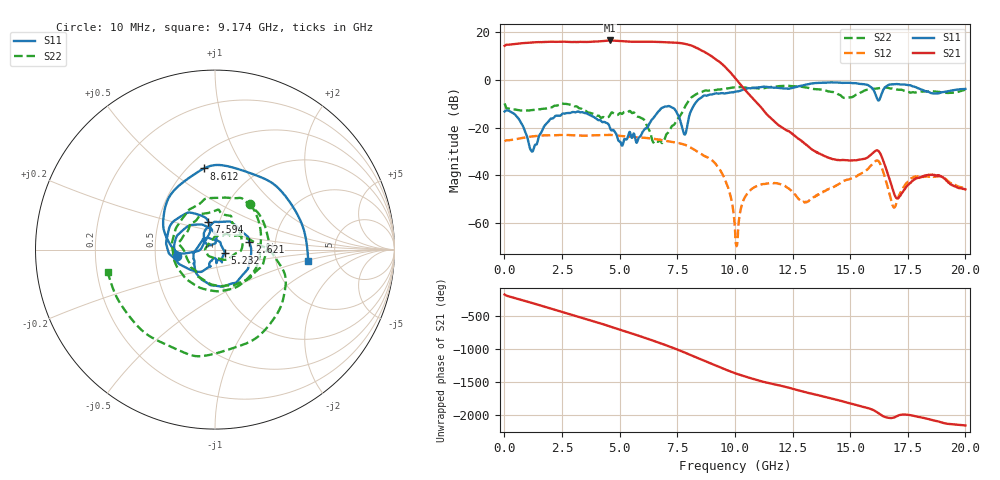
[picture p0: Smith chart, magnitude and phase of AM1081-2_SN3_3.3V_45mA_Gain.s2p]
!Agilent Technologies,E8364B,MY43040894,A.07.50.67
!Agilent E8364B: A.07.50.67
!Date: Wednesday, June 23, 2021 08:05:39
!Correction: S11(Full 2 Port(1,2))
!S21(Full 2 Port(1,2))
!S12(Full 2 Port(1,2))
!S22(Full 2 Port(1,2))
!S2P File: Measurements: S11, S21, S12, S22:
# Hz S  dB  R 50
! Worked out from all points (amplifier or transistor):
!   3201 points, 10 MHz to 20 GHz, reference 50 ohm
!   highest |S21| = 16.6 dB at 4.595 GHz (marker M1)
!   |S21| within 3 dB of that: start of sweep to 8.292 GHz
!   unconditionally stable (mu >= 1): start of sweep to end of sweep
!   at 3.34 GHz: K = 1.21, MAG = 17.0 dB, |S12| = -23.4 dB
!   at 10.01 GHz: K = 214.87, MAG = 5.5 dB, |S12| = -62.7 dB
!   at 20 GHz: K = 6787.26, MAG = -41.5 dB, |S12| = -45.6 dB
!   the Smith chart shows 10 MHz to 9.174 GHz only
!   S11 on the Smith chart (normalised r, x): 10 MHz: 0.65, -0.05; 2.621 GHz: 1.47, +0.13; 5.232 GHz: 1.11, -0.04; 7.594 GHz: 0.89, +0.28; 8.612 GHz: 0.59, +0.68; 9.174 GHz: 3.09, -0.52
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1e7  -13.25 -169.9  14.33 -169.4  -25.75 11.8  -9.86 52.2
6.221938e8  -16.34 115.7  15.30 121.3  -24.68 -46.8  -12.69 -88.1
1.078216e9  -27.72 82.6  15.65 74.8  -23.89 -86.8  -12.82 -147.2
1.846581e9  -18.10 114.3  16.01 -5.2  -23.25 -159.8  -11.96 133.6
2.621194e9  -14.15 12.6  16.06 -86.7  -23.10 125.7  -10.03 44.4
3.345831e9  -13.53 -75.0  16.02 -162.2  -23.38 55.5  -12.12 -41.9
3.883062e9  -15.58 -129.7  16.12 142.0  -23.25 4.3  -14.43 -100.5
4.264122e9  -17.74 -153.6  16.32 101.0  -23.14 -33.8  -15.58 -142.4
4.595206e9  -20.48 168.5  16.60 63.3  -23.10 -68.8  -14.53 175.5
5.232388e9  -24.80 -19.4  16.17 -9.9  -23.72 -134.8  -13.48 110.0
5.969519e9  -22.39 -112.2  16.09 -93.3  -24.23 148.2  -16.12 12.0
6.675416e9  -13.30 -158.8  15.97 -179.0  -25.02 68.5  -25.99 -162.0
7.187659e9  -11.10 144.9  15.76 115.9  -25.93 8.4  -20.83 61.5
7.593706e9  -15.97 103.5  15.52 60.8  -26.60 -42.4  -15.54 25.1
8.037234e9  -14.51 -173.3  14.65 -3.4  -28.19 -103.1  -8.12 -16.2
8.611947e9  -6.81 97.7  12.09 -88.1  -31.59 -175.3  -4.86 -86.9
9.174166e9  -5.64 -6.8  8.63 -169.7  -35.42 108.9  -4.28 -168.3
1.0005e10  -4.92 -167.6  0.92 73.1  -62.67 12.7  -3.16 65.1
1.181035e10  -3.23 -1.5  -18.25 -104.8  -43.42 -6.1  -2.74 161.6
1.334083e10  -1.49 173.4  -29.14 119.5  -49.80 87.5  -3.68 2.4
1.667042e10  -2.05 12.2  -40.60 113.3  -46.53 114.1  -3.37 -84.4
2e10  -3.77 111.4  -45.95 -2.4  -45.64 -6.7  -4.15 -134.7
